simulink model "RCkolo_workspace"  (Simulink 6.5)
settings: Solver=ode45  StartTime=0.0  StopTime=1  RelTol=1e-3
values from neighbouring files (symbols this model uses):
  A = [-R/L -1/L; 1/C 0]    [primer_7_4c.m]
  C = str2num(C)    [patuvacki_bran_1.m]    (also in primer_7_3.m = 0.0001; primer_7_4.m = 0.0001; primer_7_4a.m = 0.0001; primer_7_4c.m = 0.0001)
undefined symbols (not defined in the file or in its folder): B, blocks, Continuous, D, powergui, x0, ZData
libraries: powerlib x4

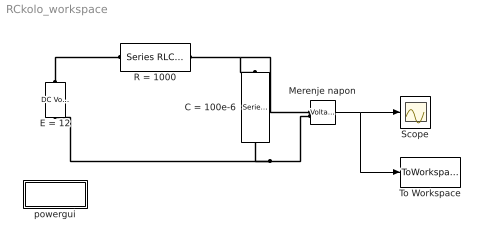
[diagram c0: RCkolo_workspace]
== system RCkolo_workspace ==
  C = 100e-6 : powerlib/Elements/Series RLC Branch  Orientation=down  DialogController=PMDialogs.PMDefaultMaskDlg  PhysicalDomain=powersysdomain  SubClassName=unknown  LeftPortType=p1  RightPortType=p1  LConnTagsString=__new0  RConnTagsString=__new0  BranchType=C  Resistance=1  Inductance=1e-3  SetiL0=off  InitialCurrent=0  Capacitance=100e-6  Setx0=on  InitialVoltage=0  Measurements=Branch voltage
  E = 12 : powerlib/Electrical Sources/DC Voltage Source  Orientation=up  DialogController=PMDialogs.PMDefaultMaskDlg  SystemSampleTime=-1  Amplitude=12  Measurements=None
  Merenje napon : powerlib/Measurements/Voltage Measurement  DialogController=PMDialogs.PMDefaultMaskDlg  SystemSampleTime=-1  PhasorSimulation=off  OutputType=Complex  PSBequivalent=0
  R = 1000 : powerlib/Elements/Series RLC Branch  DialogController=PMDialogs.PMDefaultMaskDlg  PhysicalDomain=powersysdomain  SubClassName=unknown  LeftPortType=p1  RightPortType=p1  LConnTagsString=__new0  RConnTagsString=__new0  BranchType=R  Resistance=1000  Inductance=1e-3  SetiL0=off  InitialCurrent=0  Capacitance=100e-6  Setx0=on  InitialVoltage=0  Measurements=Branch current
  Scope : Scope
  To Workspace : ToWorkspace  VariableName=u  SampleTime=-1  SaveFormat=Array
  powergui : Subsystem  AncestorBlock=powerlib/powergui  InitFcn=powergui( 'InitFcn_Callback' , gcb , 0 , [ ] );  mask(PSB option menu block){SimulationMode=Continuous, SampleTime=50e-6, echomessages=off, RestoreLinks=warning, x0status=blocks, Frange=[0:2:500], Ylog=off, Xlog=on, ShowGrid=off, save=off, variable=ZData, structure=, ZoomFFT=on, StartTime=0.0, cycles=1, DisplayStyle=1, fundamental=60, FreqAxis=off, MaxFrequency=1000, frequencyindice=0, frequencyindicesteady=1, RmsSteady=1, display=off, Ts=0, frequency=60, methode=off, HookPort=off, Interpol=off}
      mask prompts: SimulationMode "Simulation mode"; SampleTime "Sample time Ts (when simulation mode is Discrete) (s)"; echomessages "Echo  Messages"; RestoreLinks "Restore disabled links"; x0status "Initial electrical states status"; Frange "Impedance tool: Frequency Range"; Ylog "Impedance tool: Log impedance"; Xlog "Impedance tool: log Frequency"; ShowGrid "Impedance tool: grid"; save "Impedance tool: Save Data To Workspace"; variable "Impedance tool: Variable Name"; structure "Structure Name (PSBFFTSCOPE)"; ZoomFFT "ZoomFFT (PSBFFTSCOPE)"; StartTime "Start Time (PSBFFTSCOPE)"; cycles "Cycles (PSBFFTSCOPE)"; DisplayStyle "Display style (PSBFFTSCOPE)"; fundamental "Fundamental (PSBFFTSCOPE)"; FreqAxis "Frequency Axis (PSBFFTSCOPE)"; MaxFrequency "Max Frequency (PSBFFTSCOPE)"; frequencyindice "Load flow frequency (Hz)"; frequencyindicesteady "Frequency indice (STEADYSTATE)"; RmsSteady "RMS display (STEADYSTATE)"; display "Display Results"; Ts "OBSOLETE 1"; frequency "Phasor frequency (Hz)"; methode "Phasor simulation"; HookPort "Hook port"; Interpol "Interpolate"
      mask init:
      | powerlibroot = which('powersysdomain');
      | PSBroot = powerlibroot(1:end-16);
      | %
      | switch SimulationMode
      | 	case 1
      | 		message=sprintf('Continuous');
      | 	case 2
      |         SampleTimeeval=evalin('base',SampleTime,'NaN');
      |         if isnan(SampleTimeeval)
      |             message=sprintf('Warning !!,\nUndefined sample time');
      |         else
      |             message=sprintf('Discrete,\nTs = %.4g s.',SampleTimeeval);
      |         end
      | 	case 3
      | 		message=sprintf('Phasors');
      | end
      | if strcmp(bdroot,'powerlib')
      |   message='powergui';
      | end
      | power_initmask();
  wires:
  Merenje napon/1 -> To Workspace/1, Scope/1
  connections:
  E = 12/RConn1 -- R = 1000/LConn1
  R = 1000/RConn1 -- Merenje napon/LConn1 -- C = 100e-6/LConn1
  Merenje napon/LConn2 -- E = 12/LConn1 -- C = 100e-6/RConn1

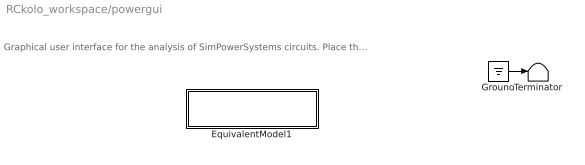
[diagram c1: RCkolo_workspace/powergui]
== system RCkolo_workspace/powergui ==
  note: Graphical user interface for the analysis of SimPowerSystems circuits. Place the Powergui block in the top-level of your model and double-click on it to open the GUI.
  EquivalentModel1 : Subsystem
  Ground : Ground
  Terminator : Terminator
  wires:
  Ground/1 -> Terminator/1

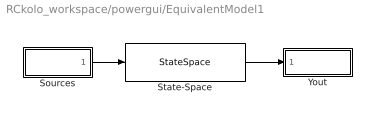
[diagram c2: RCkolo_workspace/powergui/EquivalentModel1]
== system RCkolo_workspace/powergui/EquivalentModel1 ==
  Sources : Subsystem
  State-Space : StateSpace  A=A  B=B  C=C  D=D  X0=x0
  Yout : Subsystem
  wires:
  Sources/1(u) -> State-Space/1
  State-Space/1 -> Yout/1(v,i)

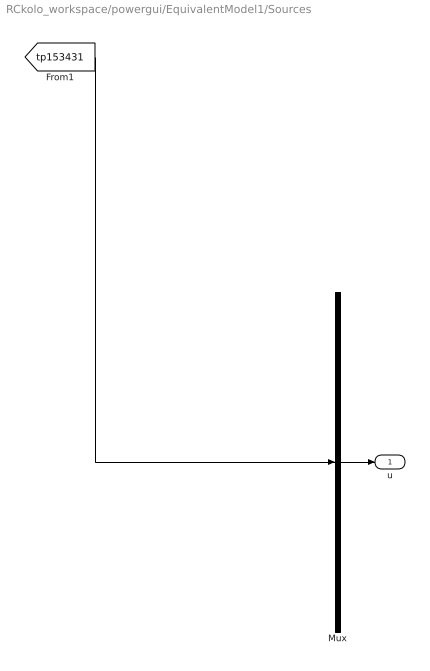
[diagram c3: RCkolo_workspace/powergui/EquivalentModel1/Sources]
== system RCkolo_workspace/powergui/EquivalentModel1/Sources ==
  Mux : Mux  Inputs=1
  u : Outport
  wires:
  Mux/1 -> u/1
  [tp153431] -> Mux/1

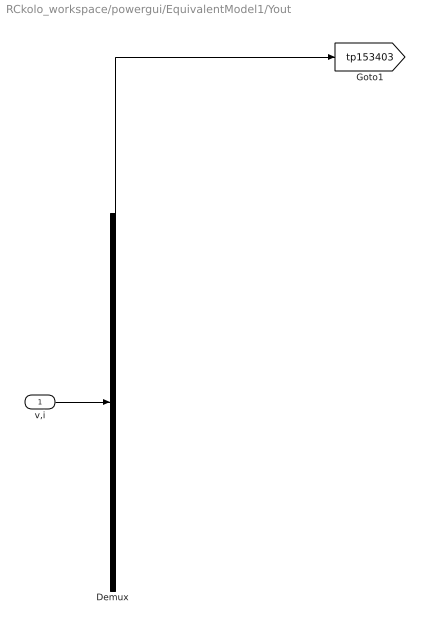
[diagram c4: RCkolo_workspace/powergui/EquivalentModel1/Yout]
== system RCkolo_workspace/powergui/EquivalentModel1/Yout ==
  v,i : Inport
  Demux : Demux  Outputs=1
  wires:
  v,i/1 -> Demux/1
  Demux/1 -> [tp153403]
